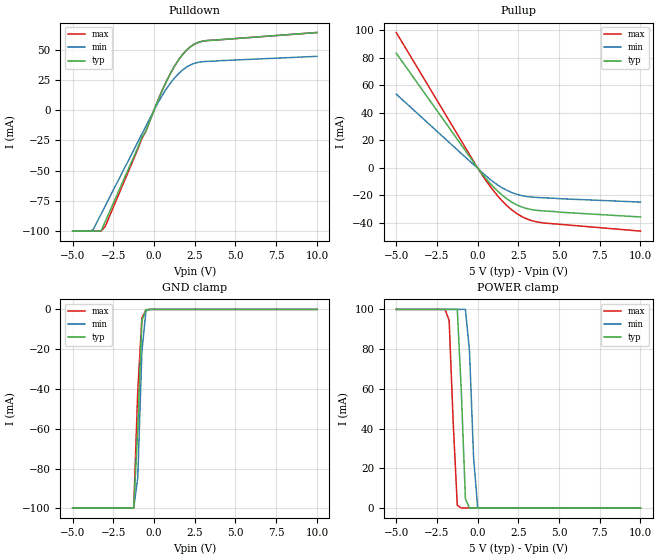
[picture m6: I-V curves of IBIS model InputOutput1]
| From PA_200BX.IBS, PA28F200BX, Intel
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|********************Input Output Model 1*****************************
[Model]   InputOutput1
Model_type   I/O
|   Model for: DQ[0:14].
Vinl = 0.8V
Vinh = 2.0V
|Variable   typ   min   max
C_comp   8.91p   NA   10.5p
[Voltage Range]   5.0V   4.5V   5.5V
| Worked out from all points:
|   slope of the pulldown table from 0 to 0.75 V, typ, clamps not added: 31.9 ohm
|   slope of the pullup table from 0 to 0.75 V, typ, clamps not added: 68.4 ohm
|   GND clamp passes 1 mA (typ) near -0.54 V on its own axis
|   POWER clamp passes 1 mA (typ) near -0.55 V on its own axis
[Pulldown]
| [Pullup] and [Pulldown] IV curves include only the current through
| the channels of output driver transistors when outputs are enabled
| with OE# = VIL.  Although the output driver transistors have np and
| pn diodes inherently created by CMOS IC fabrication between the
| drain and bulk of n-channel and p-channel CMOS transistors,
| the current through these junction diodes is not included in
| [Pullup] or [Pulldown].  Instead that drain/bulk diode current is
| included in the [POWER_clamp] or [GND_clamp] sections, which are
| not dependent on the state of OE# or output data value.
|Voltage   I(typ)   I(min)   I(max)
-5V       -100mA     -100mA     -100mA
-3.75V    -100mA     -98.99mA   -100mA
-3.25V    -99.73mA   -85.79mA   -100mA
-3V       -92.1mA    -79.19mA   -96.1mA
-750mV    -22.49mA   -19.79mA   -23.66mA
-500mV    -17.35mA   -13.19mA   -17.33mA
500mV     16.24mA    12.09mA    16.24mA
1V        30.19mA    22.18mA    30.19mA
1.5V      41.41mA    30.06mA    41.41mA
2.25V     52.52mA    37.45mA    52.52mA
3.25V     57.46mA    40.25mA    57.46mA
10V       64.1mA     44.4mA     64.1mA
[GND_clamp]
| [POWER_clamp] and [GND_clamp] IV curves describe ESD protection
| circuits PLUS some np and pn diodes which exist between the
| drain and bulk of n-channel and p-channel CMOS transistors.
| These drain/bulk diodes are inherent in CMOS IC fabrication,
| and are visible on the node of the I/O pin at all times.
| Even the drain/bulk diodes of output driver [Pullup] and [Powerdown]
| transistors are included in [POWER_clamp] or [GND_clamp], because
| these diodes contribute to I/O pin current even when the
| chip outputs are tristated by OE# = VIH.
| For example, when V forced on the I/O pin is large, we are
| forward biasing the pn diode at the drain/bulk interface in the
| p-channel pullup transistor.  Similarly, when V forced on the
| I/O pin is sufficiently negative with respect to the substrate
| ground, we are forward biasing the np diode at the drain/bulk
| interface in the n-channel pulldown transistor.  The effects
| of these diodes are included in [POWER_clamp] or [GND_clamp].
|Voltage   I(typ)   I(min)   I(max)
-5V       -99.85mA   -99.85mA   -99.85mA
-1.25V    -99.85mA   -99.85mA   -99.85mA
-1V       -60mA      -84.53mA   -40.79mA
-750mV    -5.562mA   -21.29mA   -4.395mA
-500mV    -191.4uA   -722.8uA   -214.3uA
-250mV    -32.36nA   -2.075uA   -15.38nA
10V       0A         0A         0A
[Pullup]
| (Voltages for [Pullup] and [POWER_clamp] are specified with
| negative respect to Vcc.  Reference the IBIS documentation
| for more information regarding Vtable = Vcc - Voutput.
| This method keeps -Vds constant for the values in all three
| columns across a line of the table.
| [Pullup] and [Pulldown] IV curves include only the current through
| the channels of output driver transistors when outputs are enabled
| with OE# = VIL.  Although the output driver transistors have np and
| pn diodes inherently created by CMOS IC fabrication between the
| drain and bulk of n-channel and p-channel CMOS transistors,
| the current through these junction diodes is not included in
| [Pullup] or [Pulldown].  Instead that drain/bulk diode current is
| included in the [POWER_clamp] or [GND_clamp] sections, which are
| not dependent on the state of OE# or output data value.
|Voltage  I(typ)   I(min)   I(max)
-5V       83.48mA    53.7mA     98.47mA
250mV     -3.874mA   -2.949mA   -4.576mA
750mV     -10.96mA   -8.165mA   -13.07mA
1.25V     -17.05mA   -12.53mA   -20.57mA
2V        -24.1mA    -17.39mA   -29.52mA
2.75V     -28.52mA   -20.19mA   -35.55mA
3.25V     -30.11mA   -21.06mA   -38.01mA
3.75V     -30.93mA   -21.51mA   -39.43mA
10V       -35.6mA    -24.8mA    -45.9mA
[POWER_clamp]
| (Voltages for [Pullup] and [POWER_clamp] are specified with
| negative respect to Vcc.  Reference the IBIS documentation
| for more information regarding Vtable = Vcc - Voutput.
| This method keeps -Vds constant for the values in all three
| columns across a line of the table.
| [POWER_clamp] and [GND_clamp] IV curves describe ESD protection
| circuits PLUS some np and pn diodes which exist between the
| drain and bulk of n-channel and p-channel CMOS transistors.
| These drain/bulk diodes are inherent in CMOS IC fabrication,
| and are visible on the node of the I/O pin at all times.
| Even the drain/bulk diodes of output driver [Pullup] and [Powerdown]
| transistors are included in [POWER_clamp] or [GND_clamp], because
| these diodes contribute to I/O pin current even when the
| chip outputs are tristated by OE# = VIH.
| For example, when V forced on the I/O pin is large, we are
| forward biasing the pn diode at the drain/bulk interface in the
| p-channel pullup transistor.  Similarly, when V forced on the
| I/O pin is sufficiently negative with respect to the substrate
| ground, we are forward biasing the np diode at the drain/bulk
| interface in the n-channel pulldown transistor.  The effects
| of these diodes are included in [POWER_clamp] or [GND_clamp].
|Voltage I(typ)   I(min)   I(max)
-5V       100mA      100mA      100mA
-2V       100mA      100mA      100mA
-1.75V    100mA      100mA      94.44mA
-1.5V     100mA      100mA      42.84mA
-1.25V    100mA      100mA      1.343mA
-1V       58.11mA    100mA      40.86nA
-750mV    4.582mA    100mA      0A
-500mV    543.5nA    79.07mA    0A
-250mV    0A         25.67mA    0A
0V        0A         242.8uA    0A
10V       0A         0A         0A
[Ramp]
| The DQ Ramp information is not provided at this time for the
| device but will be available in the future.  The table below
| is for the compatibility with some IBIS parsers.
| Variable   typ   min   max
 dV/dt_r   0V/0ns   0V/0ns   0V/0ns
 dV/dt_f   0V/0ns   0V/0ns   0V/0ns
